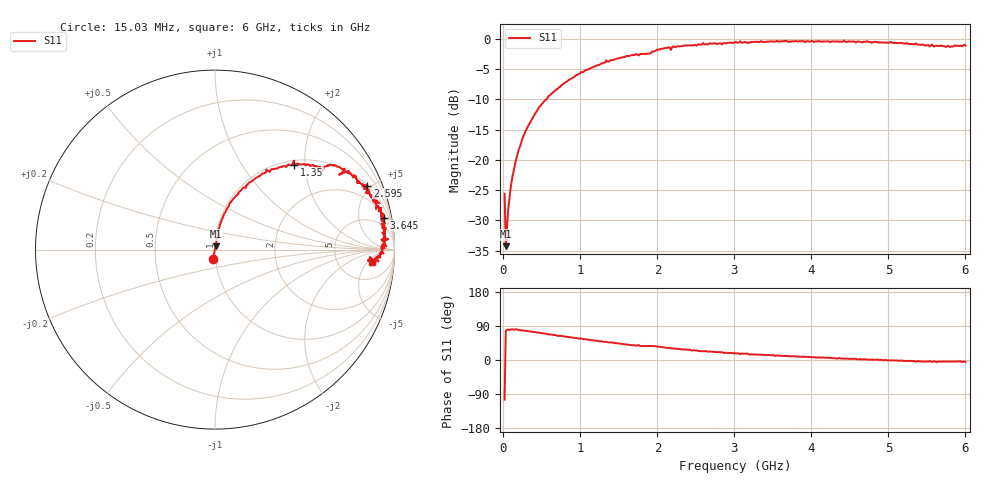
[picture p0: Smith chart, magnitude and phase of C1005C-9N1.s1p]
!	Network	Analyzer	HP8753E.07.74:	Oct	30	2002	Serial	No.	JP38451487
!	Hewlett-Packard
!	28	Aug	2009	9:01:33
!	Frequency	S11
#	HZ	S	RI	R	50
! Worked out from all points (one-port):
!   400 points, 15.03 MHz to 6 GHz, reference 50 ohm
!   lowest |S11| = -34.3 dB at 30.03 MHz (marker M1), VSWR 1.04, Z = 50.4 + j1.9 ohm
!   |S11| at or under -10 dB: start of sweep to 559.3 MHz
!   S11 on the Smith chart (normalised r, x): 15.03 MHz: 0.97, -0.10; 1.35 GHz: 1.08, +1.76; 2.595 GHz: 1.02, +4.74; 3.645 GHz: 2, +10; 6 GHz: 11, -7
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1.502992e7  -0.0132 -0.0507
3.002985e7  0.00445 0.0188
6.00297e7  0.00644 0.0372
1.050295e8  0.0107 0.0645
1.650292e8  0.0152 0.0995
2.550287e8  0.0324 0.151
4.650277e8  0.0822 0.261
7.650262e8  0.188 0.372
1.005025e9  0.286 0.446
1.350023e9  0.44 0.474
1.515022e9  0.506 0.47
2.02502e9  0.67 0.47
2.145019e9  0.722 0.451
2.175019e9  0.691 0.417
2.205019e9  0.747 0.437
2.265019e9  0.754 0.426
2.595017e9  0.848 0.357
2.835016e9  0.84 0.317
3.015015e9  0.897 0.289
3.195014e9  0.897 0.226
3.645012e9  0.943 0.178
3.765011e9  0.935 0.164
4.515007e9  0.946 0.0562
5.265004e9  0.908 -0.0432
5.535002e9  0.862 -0.0426
5.625002e9  0.87 -0.0884
5.745001e9  0.852 -0.0604
6e9  0.877 -0.07
